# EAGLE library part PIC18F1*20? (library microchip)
18/20/28-Pin High-Performance, Enhanced Flash Microcontrollers with 10-bit A/D and nanoWatt Technology Source: ww1.microchip.com/downloads/en/DeviceDoc/39605c.pdf
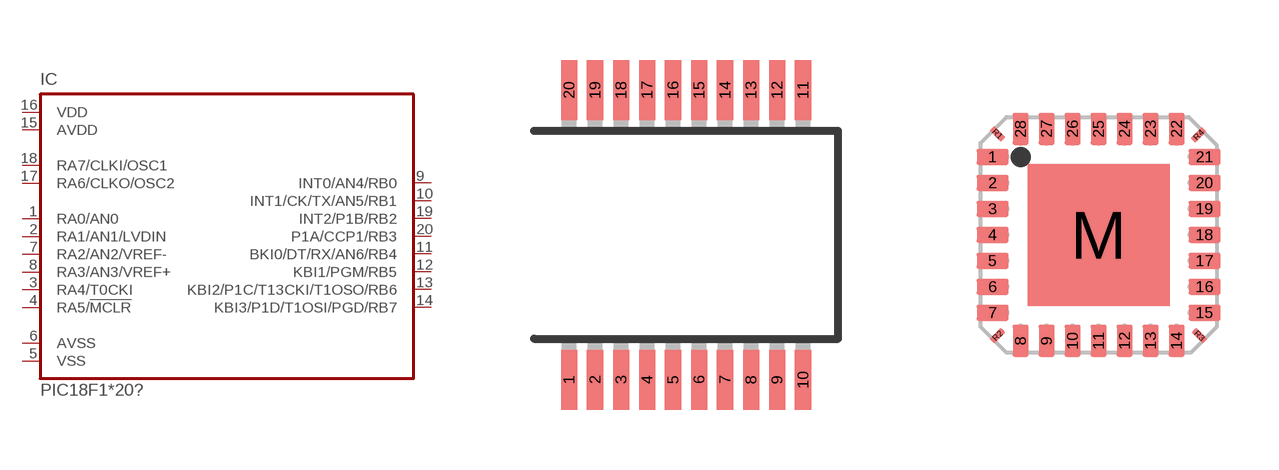
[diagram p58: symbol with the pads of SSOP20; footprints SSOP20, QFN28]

Designator prefix IC

## PIC18F1220SS (MF: MICROCHIP; MPN: PIC18F1220-E/SS; OC_FARNELL: 9761993; OC_NEWARK: 92C4995), PIC18F1320SS (MF: MICROCHIP; MPN: PIC18F1320-I/SS; OC_FARNELL: 1084333; OC_NEWARK: 92C5009)  [SSOP20]
1  RA0/AN0
2  RA1/AN1/LVDIN
3  RA4/T0CKI
4  RA5/!MCLR  in
5  VSS  pwr
6  AVSS  pwr
7  RA2/AN2/VREF-
8  RA3/AN3/VREF+
9  INT0/AN4/RB0
10  INT1/CK/TX/AN5/RB1
11  BKI0/DT/RX/AN6/RB4
12  KBI1/PGM/RB5
13  KBI2/P1C/T13CKI/T1OSO/RB6
14  KBI3/P1D/T1OSI/PGD/RB7
15  AVDD  pwr
16  VDD  pwr
17  RA6/CLKO/OSC2
18  RA7/CLKI/OSC1
19  INT2/P1B/RB2
20  P1A/CCP1/RB3

## PIC18F1220ML (MF: MICROCHIP; MPN: PIC18F1220-I/ML; OC_FARNELL: unknown; OC_NEWARK: 92C4996), PIC18F1320ML (MF: MICROCHIP; MPN: PIC18F1320-I/ML; OC_FARNELL: 9762000; OC_NEWARK: 92C5008)  [QFN28]
1  RA5/!MCLR  in
3  VSS  pwr
5  AVSS  pwr
7  RA2/AN2/VREF-
8  RA3/AN3/VREF+
9  INT0/AN4/RB0
10  INT1/CK/TX/AN5/RB1
12  BKI0/DT/RX/AN6/RB4
13  KBI1/PGM/RB5
15  KBI2/P1C/T13CKI/T1OSO/RB6
16  KBI3/P1D/T1OSI/PGD/RB7
17  AVDD  pwr
19  VDD  pwr
20  RA6/CLKO/OSC2
21  RA7/CLKI/OSC1
23  INT2/P1B/RB2
24  P1A/CCP1/RB3
26  RA0/AN0
27  RA1/AN1/LVDIN
28  RA4/T0CKI

## Footprint SSOP20 (pad centres in mm)
Shrink Small Outline Package package type SS
smd 0.4 x 1.5: 1 -2.925,-3.625; 2 -2.275,-3.625; 3 -1.625,-3.625; 4 -0.975,-3.625; 5 -0.325,-3.625; 6 0.325,-3.625; 7 0.975,-3.625; 8 1.625,-3.625; 9 2.275,-3.625; 10 2.925,-3.625; 11 2.925,3.625; 12 2.275,3.625; 13 1.625,3.625; 14 0.975,3.625; 15 0.325,3.625; 16 -0.325,3.625; 17 -0.975,3.625; 18 -1.625,3.625; 19 -2.275,3.625; 20 -2.925,3.625

## Footprint QFN28 (pad centres in mm)
28-Lead Plastic Quad Flat No Lead Package (ML) 6x6 mm Body, Punch Singulated (QFN) Source: ww1.microchip.com/downloads/en/DeviceDoc/39605c.pdf
smd 0.8 x 0.4: 1 -2.65,1.95; 2 -2.65,1.3; 3 -2.65,0.65; 4 -2.65,0; 5 -2.65,-0.65; 6 -2.65,-1.3; 7 -2.65,-1.95; 15 2.65,-1.95; 16 2.65,-1.3; 17 2.65,-0.65; 18 2.65,0; 19 2.65,0.65; 20 2.65,1.3; 21 2.65,1.95
smd 0.4 x 0.8: 8 -1.95,-2.65; 9 -1.3,-2.65; 10 -0.65,-2.65; 11 0,-2.65; 12 0.65,-2.65; 13 1.3,-2.65; 14 1.95,-2.65; 22 1.95,2.65; 23 1.3,2.65; 24 0.65,2.65; 25 0,2.65; 26 -0.65,2.65; 27 -1.3,2.65; 28 -1.95,2.65
smd 3.55 x 3.55: M 0,0
smd 0.17 x 0.4 rotated 45: R1 -2.525,2.525
smd 0.17 x 0.4 rotated 135: R2 -2.525,-2.525
smd 0.17 x 0.4 rotated 225: R3 2.525,-2.525
smd 0.17 x 0.4 rotated 315: R4 2.5,2.5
